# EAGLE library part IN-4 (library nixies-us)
IN-4: large numeric topview nixie tube
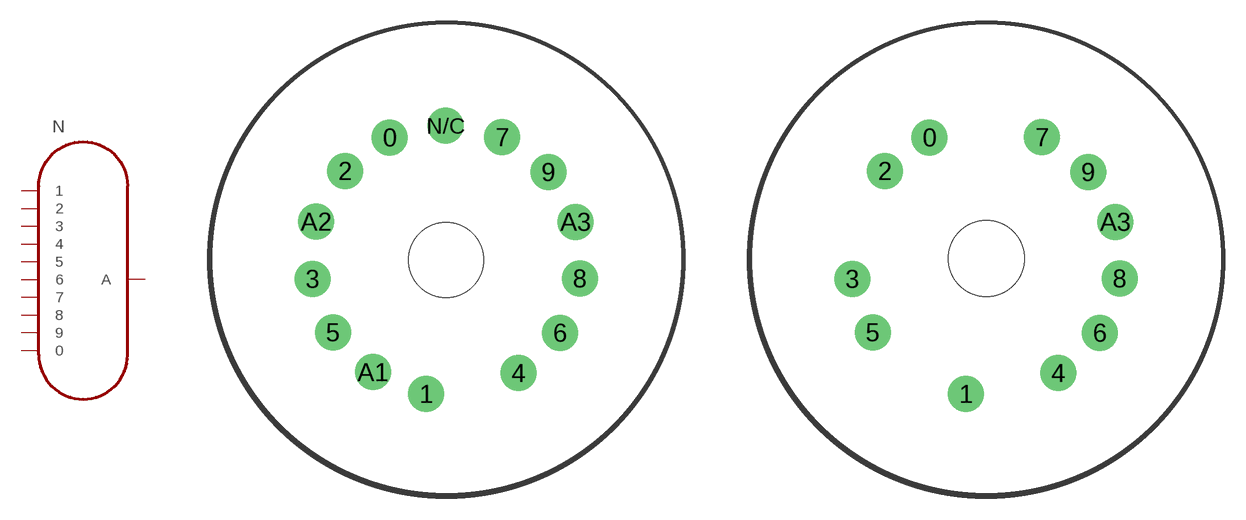
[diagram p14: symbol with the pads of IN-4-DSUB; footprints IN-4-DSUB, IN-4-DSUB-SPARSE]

Designator prefix N

## IN-4  [IN-4-DSUB]
0  0
1  1
2  2
3  3
4  4
5  5
6  6
7  7
8  8
9  9
A3  A

## IN-4SPARSE  [IN-4-DSUB-SPARSE]
Pads as for IN-4-DSUB

## Footprint IN-4-DSUB (pad centres in mm)
May be used with socket: PL31-P
drill 1.6: 0 -3.793,8.084; 1 -1.363,-9.027; 2 -6.784,5.848; 3 -8.938,-1.353; 4 4.793,-7.632; 5 -7.577,-4.914; 6 7.547,-4.945; 7 3.707,8.102; 8 8.878,-1.322; 9 6.789,5.777; A1 -4.919,-7.571; A2 -8.707,2.468; A3 8.601,2.454; N/C -0.063,8.869
hole 5 at -0.033,-0.087

## Footprint IN-4-DSUB-SPARSE (pad centres in mm)
May be used with socket: PL31-P
drill 1.6: 0 -3.793,8.084; 1 -1.363,-9.027; 2 -6.784,5.848; 3 -8.938,-1.353; 4 4.793,-7.632; 5 -7.577,-4.914; 6 7.547,-4.945; 7 3.707,8.102; 8 8.878,-1.322; 9 6.789,5.777; A3 8.601,2.454
hole 5.08 at 0,0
